FUNCTION "ZWPH" : VOID
TITLE =
AUTHOR : WE_ZA
FAMILY : Regeln
NAME : ZWPH
VERSION : 0.1


VAR_INPUT
  EIN : BOOL ;
  SW : REAL ;
  IW : REAL ;
  SH : REAL ;
END_VAR
VAR_OUTPUT
  STG : BOOL ;
END_VAR
VAR_TEMP
  ER : REAL ;
  SP : REAL ;
END_VAR
BEGIN
NETWORK
TITLE =

      UN    #EIN;
      R     #STG;
      BEB   ;
      L     #SW;
      L     #IW;
      -R    ;
      T     #ER;
      L     5.000000e-003;
      L     #SH;
      *R    ;
      L     #SW;
      *R    ;
      T     #SP;
      L     #ER;
      L     #SP;
      >R    ;
      S     #STG;
      BEB   ;
      L     #SP;
      L     -1.000000e+000;
      *R    ;
      L     #ER;
      TAK   ;
      <R    ;
      R     #STG;






END_FUNCTION

